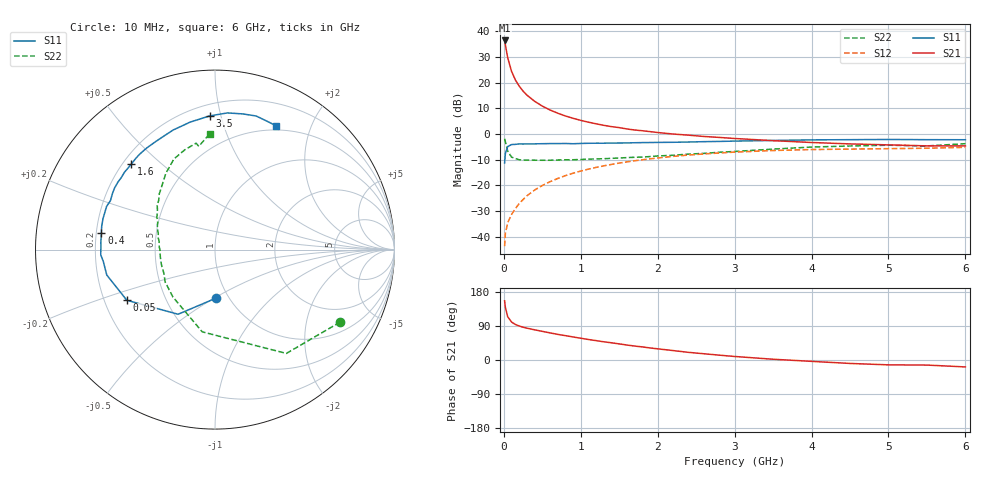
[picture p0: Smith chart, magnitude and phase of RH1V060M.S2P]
! SIEMENS Small Signal Semiconductors
! BFR106
! Si NPN RF Bipolar Junction Transistor in SOT23
! VCE = 1 V  IC = 60 mA
! Common Emitter S-Parameters:  August  1996
# GHz  S  MA  R  50
!  f  S11  S21  S12  S22
! GHz  MAG  ANG  MAG  ANG  MAG  ANG  MAG  ANG
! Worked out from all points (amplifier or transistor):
!   36 points, 10 MHz to 6 GHz, reference 50 ohm
!   highest |S21| = 36.4 dB at 10 MHz (marker M1)
!   |S21| within 3 dB of that: start of sweep to 27.66 MHz
!   unconditionally stable (mu >= 1): 166.4 MHz to end of sweep
!   at 250 MHz: K = 1.08, MAG = 19.4 dB, |S12| = -25.6 dB
!   at 1.4 GHz: K = 1.09, MAG = 5.5 dB, |S12| = -11.9 dB
!   at 6 GHz: K = 1.03, MAG = -0.8 dB, |S12| = -5.2 dB
!   S11 on the Smith chart (normalised r, x): 10 MHz: 0.87, -0.51; 50 MHz: 0.29, -0.25; 400 MHz: 0.22, +0.07; 1.6 GHz: 0.23, +0.40; 3.5 GHz: 0.28, +0.92; 6 GHz: 0.45, +1.51
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0.01  0.2717 -89.4  66.09 156.1  0.0065 71.8  0.8056 -30.1
0.02  0.4146 -119.7  54.18 138.9  0.0115 60.4  0.7019 -55.5
0.05  0.5666 -150.1  30.5 114.2  0.0186 54.3  0.4637 -98.8
0.1  0.6194 -166.8  16.58 100.2  0.0269 59.0  0.3531 -131.6
0.15  0.6255 -173.8  11.23 93.8  0.035 63.5  0.3311 -146.9
0.2  0.6371 -177.4  8.522 89.7  0.044 67.4  0.3135 -155.5
0.25  0.636 179.0  6.808 86.5  0.0527 68.3  0.3106 -162.1
0.3  0.6374 176.2  5.699 84.0  0.0623 69.7  0.3094 -165.9
0.4  0.6398 171.8  4.318 79.7  0.0806 70.3  0.3073 -172.2
0.5  0.6443 168.5  3.479 75.6  0.0988 69.8  0.3065 -176.6
0.6  0.6474 164.6  2.923 71.6  0.1172 68.8  0.3066 -179.6
0.7  0.648 160.9  2.53 67.6  0.1352 67.7  0.3103 177.8
0.9  0.6432 154.9  2.013 60.8  0.1715 64.4  0.3137 172.3
1.1  0.6564 148.5  1.689 54.1  0.2059 61.2  0.3225 168.5
1.3  0.6584 142.5  1.468 48.0  0.2388 57.4  0.3286 164.1
1.6  0.6669 134.3  1.247 39.5  0.2852 51.8  0.3451 158.4
2.2  0.6865 118.9  0.994 24.9  0.3646 40.7  0.3832 146.7
2.8  0.7132 104.9  0.854 12.8  0.4244 30.0  0.439 135.0
3.5  0.7454 92.3  0.738 2.0  0.4747 18.9  0.5055 122.8
4.5  0.7717 78.4  0.638 -9.1  0.5057 5.2  0.581 106.8
5.5  0.7717 67.8  0.584 -13.4  0.5257 -2.7  0.5827 98.9
6  0.7693 63.9  0.583 -18.3  0.5474 -9.1  0.6449 92.7
